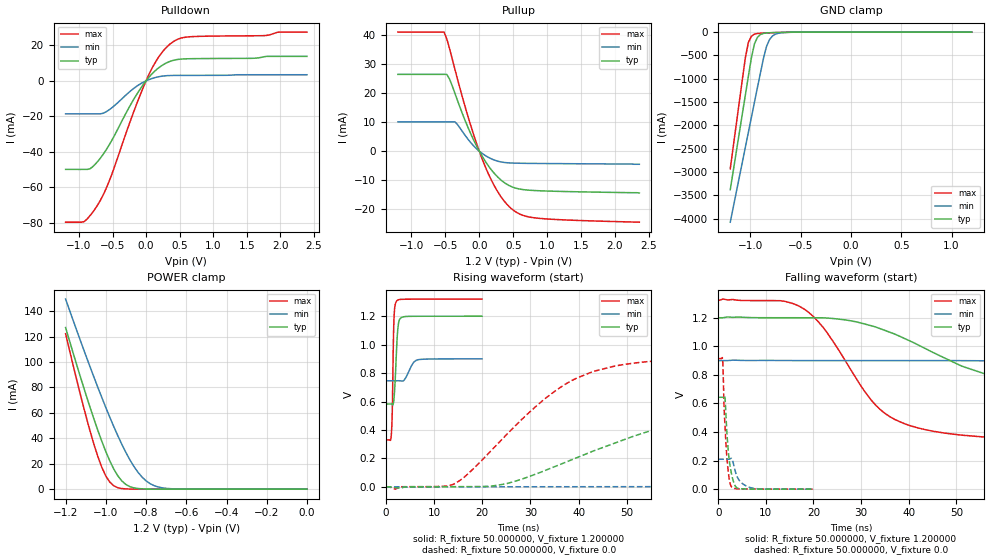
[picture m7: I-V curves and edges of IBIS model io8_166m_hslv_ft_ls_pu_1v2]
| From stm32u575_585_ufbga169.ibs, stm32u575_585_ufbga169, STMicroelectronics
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|   Model io8_166m_hslv_ft_ls_pu_1v2
[Model]  io8_166m_hslv_ft_ls_pu_1v2
Model_type I/O
Polarity   Non-Inverting
Enable   Active-Low
Vinl =   0.360000V
Vinh =   0.840000V
Vmeas =  0.600000V
Cref =   50.000000pF
Rref =   100.000000M
Vref =   0.0V
C_comp   3.151600pF   3.087200pF   3.197800pF
[Temperature Range]   25.000000   0.140000k   -40.000000
[Pullup Reference]   1.200000V   0.900000V   1.320000V
[Pulldown Reference]   0.0V   0.0V   0.0V
[POWER Clamp Reference]   1.200000V   0.900000V   1.320000V
[GND Clamp Reference]   0.0V   0.0V   0.0V
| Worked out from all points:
|   slope of the pulldown table from 0 to 0.18 V, typ, clamps not added: 25.4 ohm
|   slope of the pullup table from 0 to 0.18 V, typ, clamps not added: 27.8 ohm
|   GND clamp passes 1 mA (typ) near -0.51 V on its own axis
|   POWER clamp passes 1 mA (typ) near -0.86 V on its own axis
|   rising waveform, R_fixture 50.000000, V_fixture 1.200000: 20-80 % time 537ps typ, 1.37ns min, 302ps max; typ from 0.583 V to 1.2 V
|   rising waveform, R_fixture 50.000000, V_fixture 0.0: 20-80 % time 35.4ns typ, 88.5ns min, 17.9ns max; typ from 0 V to 0.643 V
|   falling waveform, R_fixture 50.000000, V_fixture 1.200000: 20-80 % time 31.1ns typ, 74.1ns min, 12.9ns max; typ from 1.2 V to 0.583 V
|   falling waveform, R_fixture 50.000000, V_fixture 0.0: 20-80 % time 1.03ns typ, 1.72ns min, 822ps max; typ from 0.643 V to 0 V
[Pulldown]
|Voltage   I(typ)   I(min)   I(max)
-1.2V     -49.86mA   -18.56mA   -79.56mA
-920mV    -49.86mA   -18.56mA   -79.19mA
-840mV    -49.6mA    -18.56mA   -76.08mA
-720mV    -45.32mA   -18.56mA   -69.74mA
-560mV    -36.71mA   -16.58mA   -57.44mA
-200mV    -11.43mA   -4.738mA   -19.03mA
0V        0A         0A         0A
160mV     6.477mA    2.074mA    11.78mA
360mV     10.99mA    2.988mA    20.81mA
480mV     12.07mA    3.052mA    23.52mA
640mV     12.43mA    3.072mA    24.76mA
2.4V      13.77mA    3.423mA    27.43mA
[Pullup]
|Voltage   I(typ)   I(min)   I(max)
-1.2V     26.49mA    10.13mA    41.07mA
-520mV    26.49mA    10.13mA    41.07mA
-480mV    26.49mA    10.13mA    38.77mA
-440mV    24.94mA    10.13mA    35.49mA
-360mV    19.99mA    10.13mA    28.26mA
-160mV    7.809mA    3.929mA    11.44mA
40mV      -1.649mA   -721uA     -2.521mA
240mV     -8.14mA    -3.199mA   -12.72mA
480mV     -12.27mA   -4.076mA   -19.94mA
640mV     -13.22mA   -4.166mA   -22.09mA
880mV     -13.63mA   -4.229mA   -23.13mA
2.36V     -14.4mA    -4.5mA     -24.47mA
[GND_clamp]
|Voltage   I(typ)   I(min)   I(max)
-1.2V     -3.379A    -4.076A    -2.932A
-1.05V    -1.35A     -2.47A     -550.7mA
-1.02V    -947.8mA   -2.149A    -221.5mA
-990mV    -552.4mA   -1.829A    -88.44mA
-960mV    -255.3mA   -1.51A     -44.87mA
-930mV    -111.8mA   -1.191A    -30.68mA
-870mV    -28.36mA   -564.6mA   -21.34mA
-840mV    -18.65mA   -309.5mA   -18.49mA
-810mV    -14.07mA   -161.6mA   -15.92mA
-780mV    -11.37mA   -83.33mA   -13.53mA
-600mV    -3.009mA   -4.322mA   -3.091mA
1.2V      0A         13.65nA    0A
[POWER_clamp]
|Voltage   I(typ)   I(min)   I(max)
-1.2V     127mA      149.4mA    122.2mA
-1.12V    84.98mA    114mA      70.29mA
-1.06V    55.52mA    88.42mA    35.69mA
-1.02V    37.64mA    72.04mA    17.19mA
-1V       29.52mA    64.13mA    10.33mA
-960mV    15.7mA     48.99mA    2.596mA
-900mV    3.636mA    28.77mA    207.8uA
-840mV    502.9uA    13.24mA    43.19uA
-800mV    129uA      6.535mA    43.19uA
-740mV    26.51uA    1.726mA    43.19uA
-620mV    25.02uA    82.33uA    35.3uA
0V        0A         17.36nA    0A
[Ramp]
| variable   typ   min   max
dV/dt_r  0.38567/35.33854n   0.12547/88.39758n   0.54817/17.88270n
dV/dt_f  0.37043/31.02517n   92.29800m/74.02800n 0.59405/12.85059n
R_load = 50.000000
[Rising Waveform]
R_fixture= 50.000000
V_fixture= 1.200000
V_fixture_min= 0.900000
V_fixture_max= 1.320000
|time   V(typ)   V(min)   V(max)
0s        582.6mV    746.2mV    329.9mV
1.121ns   582.7mV    746.2mV    362mV
1.321ns   580mV      746.2mV    516.3mV
1.562ns   586.8mV    746.2mV    1.02V
1.682ns   619.6mV    746.2mV    1.177V
2.242ns   983.6mV    746.2mV    1.307V
2.643ns   1.154V     746.2mV    1.316V
3.363ns   1.193V     744.1mV    1.319V
6.406ns   1.2V       891.7mV    1.32V
19.94ns   1.2V       900mV      1.32V
[Rising Waveform]
R_fixture= 50.000000
V_fixture= 0.0
V_fixture_min= 0.0
V_fixture_max= 0.0
|time   V(typ)   V(min)   V(max)
0s        434.2uV    496uV      378.8uV
14.01ns   1.257mV    822.4uV    18.11mV
25.03ns   22.49mV    848.7uV    366.7mV
38.04ns   183.5mV    1.025mV    737.5mV
47.05ns   302.2mV    1.243mV    846mV
60.06ns   444.1mV    2.536mV    894.2mV
82.08ns   575.1mV    20.69mV    910.8mV
115.1ns   630.9mV    77.25mV    913.8mV
235.2ns   643.2mV    195.7mV    914mV
498.5ns   643.3mV    209.8mV    914mV
[Falling Waveform]
R_fixture= 50.000000
V_fixture= 1.200000
V_fixture_min= 0.900000
V_fixture_max= 1.320000
|time   V(typ)   V(min)   V(max)
0s        1.2V       900mV      1.32V
17.02ns   1.2V       900.3mV    1.281V
22.02ns   1.199V     900mV      1.133V
31.03ns   1.154V     900mV      671mV
35.04ns   1.111V     900mV      529.9mV
43.04ns   991.5mV    900mV      420.1mV
57.06ns   795.4mV    898.5mV    361.8mV
82.08ns   653.6mV    879.8mV    336.5mV
129.1ns   593.7mV    804.2mV    330mV
498.5ns   582.6mV    746.2mV    329.9mV
[Falling Waveform]
R_fixture= 50.000000
V_fixture= 0.0
V_fixture_min= 0.0
V_fixture_max= 0.0
|time   V(typ)   V(min)   V(max)
0s        643.3mV    209.8mV    914mV
920.9ps   643.6mV    209.9mV    910mV
1.241ns   649.4mV    210mV      573.7mV
1.401ns   647.1mV    210mV      461.4mV
1.722ns   457.9mV    210mV      271mV
2.162ns   251.1mV    209.8mV    109.8mV
2.763ns   112.4mV    216.2mV    17.51mV
3.804ns   12.75mV    102.2mV    3.596mV
6.286ns   1.032mV    16.83mV    1.272mV
19.94ns   434.2uV    496uV      378.8uV
